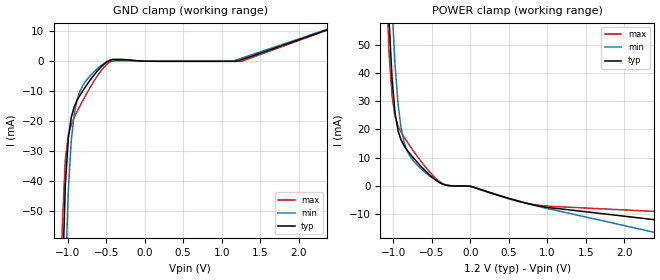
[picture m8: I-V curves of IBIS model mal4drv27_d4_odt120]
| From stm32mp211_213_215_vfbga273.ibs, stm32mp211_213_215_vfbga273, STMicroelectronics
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[Model] mal4drv27_d4_odt120
Model_type   Input
Polarity   Non-Inverting
Enable   Active-High
C_comp   1.811pF   1.688pF   1.835pF
C_comp_power_clamp   892.287fF   821.649fF   901.416fF
C_comp_gnd_clamp 799.754fF   784.236fF   811.394fF
Vinh = 771.000mV
Vinl = 656.000mV
[Model Spec]
D_overshoot_ampl_h 0.24 NA   NA
D_overshoot_ampl_l 0.24 NA   NA
D_overshoot_area_l 300.000m NA   NA
D_overshoot_area_h 300.000m NA   NA
[Receiver Thresholds]
Vth = 714.000mV
Vth_min = 678.000mV
Vth_max = 749.000mV
Vinh_ac = 68.000mV
Vinh_dc = 68.000mV
Vinl_ac = -68.000mV
Vinl_dc = -68.000mV
Tslew_ac = 5.000ns
Threshold_sensitivity = 0.5
Reference_supply Power_clamp_ref
[Temperature Range]   25.000   125.000   -40.000
[Voltage Range]   1.200V   1.140V   1.260V
[GND Clamp Reference]   0.00V   0.00V   0.00V
[C Comp Corner]
| variable   typ   min   max
C_comp 1.811pF   1.688pF   1.835pF
C_comp_pullup 892.287fF   821.649fF   901.416fF
C_comp_pulldown 799.754fF   784.236fF   811.394fF
[POWER Clamp Reference]   1.200V   1.140V   1.260V
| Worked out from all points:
|   GND clamp passes 1 mA (typ) near -0.53 V on its own axis
|   POWER clamp passes 1 mA (typ) near -0.38 V on its own axis
[GND Clamp]
-1.184V   -310.4mA   -366.8mA   -284.6mA
-1.107V   -130.1mA   -185.9mA   -102.2mA
-1.069V   -73.81mA   -120.2mA   -54.26mA
-1.031V   -41.46mA   -73.37mA   -32.9mA
-992.7mV  -25.89mA   -43.78mA   -24.81mA
-954.6mV  -18.84mA   -26.91mA   -21.17mA
-916.4mV  -15.3mA    -17.81mA   -18.8mA
-801.8mV  -9.757mA   -8.028mA   -13.06mA
-534.5mV  -1.106mA   -811uA     -2.145mA
-381.8mV  615.7uA    601.4uA    168.1uA
1.145V    163.2nA    43.22uA    9.103nA
2.367V    10.46mA    10.65mA    10.36mA
[Power Clamp]
-1.167V   165.2mA    200.8mA    149mA
-1.091V   86.82mA    121.8mA    71.56mA
-1.053V   57.74mA    89.17mA    46.31mA
-1.015V   37.55mA    62.61mA    31.63mA
-976.4mV  25.73mA    42.73mA    24.62mA
-938.2mV  19.6mA     29.2mA     21.25mA
-900mV    16.37mA    20.76mA    19.14mA
-823.6mV  12.84mA    12.68mA    15.8mA
-747.3mV  10.25mA    9.198mA    12.76mA
-365.4mV  788.7uA    940.6uA    991.1uA
856.4mV   -6.838mA   -6.96mA    -6.62mA
2.384V    -11.83mA   -16.27mA   -8.928mA
